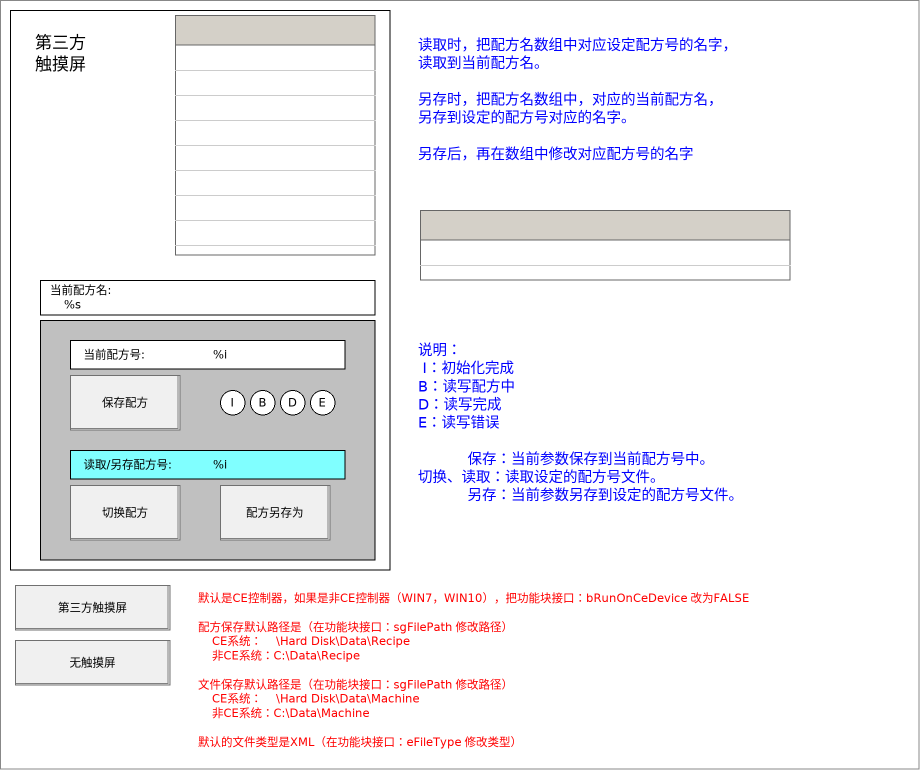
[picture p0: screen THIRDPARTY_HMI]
VISUALIZATION THIRDPARTY_HMI  // 920x770
    Rectangle (10,10 380x560), "第三方 触摸屏"
    Rectangle (40,320 335x240)
    Button (70,485 110x55), "切换配方"
        tap Recipe_OtherHMI.H_RecipeLoad
    Button (70,375 110x55), "保存配方"
        tap Recipe_OtherHMI.H_RecipeSave
    Button (220,485 110x55), "配方另存为"
        tap Recipe_OtherHMI.H_RecipeSaveAs
    Rectangle (70,340 275x29), "当前配方号:"
    Rectangle (210,340 135x29), "%i", text variable: Recipe_OtherHMI.H_CurRecipeNum
    Rectangle (70,450 275x29), "读取/另存配方号:"
    Rectangle (210,450 135x29), "%i", text variable: Recipe_OtherHMI.H_SetRecipeNum
        OnMouseDown: write the text variable via Edit
    Ellipse (250,390 25x25), "B", colour toggle: Recipe_OtherHMI.H_RecipeBusy
    Ellipse (280,390 25x25), "D", colour toggle: Recipe_OtherHMI.H_RecipeDone
    Ellipse (310,390 25x25), "E", colour toggle: Recipe_OtherHMI.H_RecipeError
    Ellipse (220,390 25x25), "I", colour toggle: Recipe_OtherHMI.H_RecipeInitialDone
    Rectangle (40,280 335x35), "当前配方名: %s", text variable: Recipe_OtherHMI.H_CurRecName
    Table (175,15 200x240), data array: Recipe_OtherHMI.H_RecipeName
        p2232123230: Recipe_OtherHMI.H_RecipeName[INDEX]
        Columns.Column.[0].Template: OnMouseDown: write the text variable via Edit
    Rectangle (415,35 375x190), "读取时，把配方名数组中对应设定配方号的名字， 读取到当前配方名。 另存时，把配方名数组中，对应的当前配方名， 另存到设定的配方号对应的名字。 另存后，再在数组中修改对应配方号的名字"
    Rectangle (415,340 375x190), "说明： I：初始化完成 B：读写配方中 D：读写完成 E：读写错误 保存：当前参数保存到当前配方号中。 切换、读取：读取设定的配方号文件。 另存：当前参数另存到设定的配方号文件。"
    Button (15,585 155x45), "第三方触摸屏"
        OnMouseClick: execute { P099_Call_Recipe.iHMI := 2; }
    Rectangle (195,590 725x180), "默认是CE控制器，如果是非CE控制器（WIN7，WIN10），把功能块接口：bRunOnCeDevice 改为FALSE 配方保存默认路径是（在功能块接口：sgFilePath 修改路径） CE系统： \Hard Disk\Data\Recipe 非CE系统：C:\Data\Recipe 文件保存默认路径是（在功能块接口：sgFilePath 修改路径） CE系统： \Hard Disk\Data\Machine 非CE系统：C:\Data\Machine 默认的文件类型是XML（在功能块接口：eFileType 修改类型）"
    Table (420,210 370x70), data array: Global_Variables_Param.sRecData
        p1755163831: rPressure
        p1791247317: Global_Variables_Param.sRecData.rPressure
        p2232123230: rSpeedRpm
        p3854506369: Global_Variables_Param.sRecData.rSpeedRpm
        p511219082: rTemp
        p1892666644: Global_Variables_Param.sRecData.rTemp
        Columns.Column.[0].Template: OnMouseDown: write the text variable via Edit
        Columns.Column.[1].Template: OnMouseDown: write the text variable via Edit
        Columns.Column.[2].Template: OnMouseDown: write the text variable via Edit
    Button (15,640 155x45), "无触摸屏"
        OnMouseClick: execute { P099_Call_Recipe.iHMI := 0; }
END_VISUALIZATION
